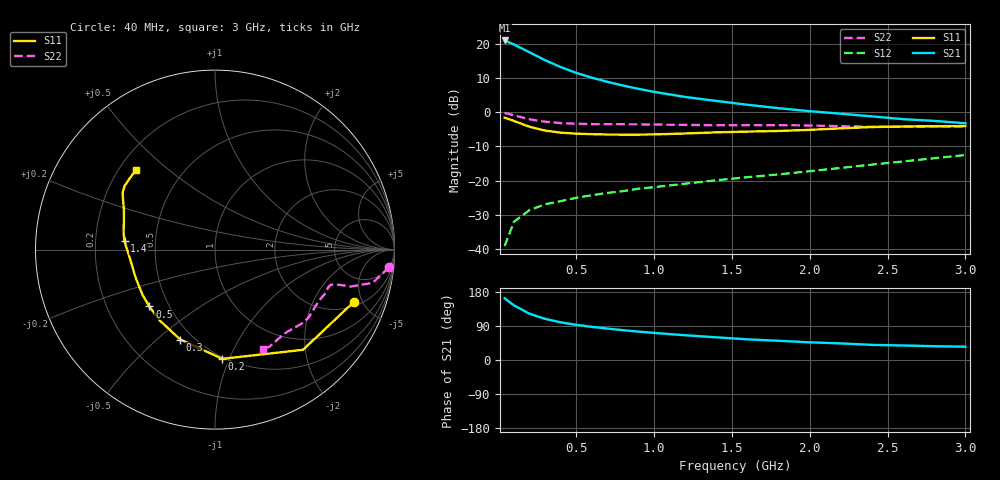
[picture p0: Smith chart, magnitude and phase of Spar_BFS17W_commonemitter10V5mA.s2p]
! Filename:  BFS17WG.S2P  Version:  4.0
! NXP part #: BFS17W  Date: Jun 1994
! Bias condition: Vce=10V, Ic=5mA
#  MHz  S  MA  R  50
! Freq  S11  S21  S12  S22  !GUM [dB]
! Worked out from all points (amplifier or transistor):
!   21 points, 40 MHz to 3 GHz, reference 50 ohm
!   highest |S21| = 20.9 dB at 40 MHz (marker M1)
!   |S21| within 3 dB of that: start of sweep to 179.8 MHz
!   unconditionally stable (mu >= 1): 597.3 MHz to end of sweep
!   at 300 MHz: K = 0.67, MSG = 21.0 dB, |S12| = -26.9 dB
!   at 1 GHz: K = 1.20, MAG = 11.2 dB, |S12| = -21.9 dB
!   at 3 GHz: K = 1.01, MAG = 3.9 dB, |S12| = -12.5 dB
!   S11 on the Smith chart (normalised r, x): 40 MHz: 2.33, -4.29; 200 MHz: 0.49, -0.94; 300 MHz: 0.42, -0.60; 500 MHz: 0.39, -0.32; 1.4 GHz: 0.33, +0.04; 3 GHz: 0.27, +0.39
40  0.827 -20.6  11.13 162.9  0.011 78.4  0.975 -5.8
100  0.743 -48.7  9.717 144.1  0.025 65.0  0.898 -11.9
200  0.61 -86.2  7.473 122.1  0.037 54.6  0.784 -15.2
300  0.537 -111.1  5.728 108.5  0.045 51.6  0.723 -15.8
400  0.501 -127.8  4.548 99.4  0.05 52.1  0.691 -16.2
500  0.484 -139.1  3.743 92.8  0.056 53.7  0.675 -16.9
600  0.476 -147.9  3.185 87.5  0.061 55.7  0.667 -17.9
700  0.47 -154.8  2.767 82.9  0.066 57.8  0.664 -18.8
800  0.469 -160.7  2.444 78.7  0.07 59.9  0.663 -19.8
900  0.469 -165.9  2.186 74.9  0.076 61.8  0.662 -20.8
1000  0.472 -170.7  1.975 71.5  0.08 63.5  0.66 -21.9
1200  0.487 -178.9  1.664 65.3  0.09 66.9  0.65 -24.7
1400  0.506 174.8  1.455 59.8  0.101 70.5  0.643 -28.5
1600  0.519 169.2  1.28 54.5  0.112 73.9  0.643 -32.8
1800  0.53 163.3  1.14 50.7  0.123 77.5  0.644 -36.3
2000  0.55 157.2  1.031 46.6  0.137 80.9  0.638 -39.8
2200  0.579 152.1  0.947 43.8  0.153 83.7  0.622 -44.1
2400  0.605 148.3  0.866 39.8  0.171 85.8  0.608 -49.8
2600  0.616 144.8  0.788 38.3  0.19 87.1  0.611 -55.8
2800  0.619 140.1  0.744 36.4  0.212 88.5  0.62 -60.5
3000  0.626 134.7  0.686 35.1  0.236 89.3  0.618 -64.2
